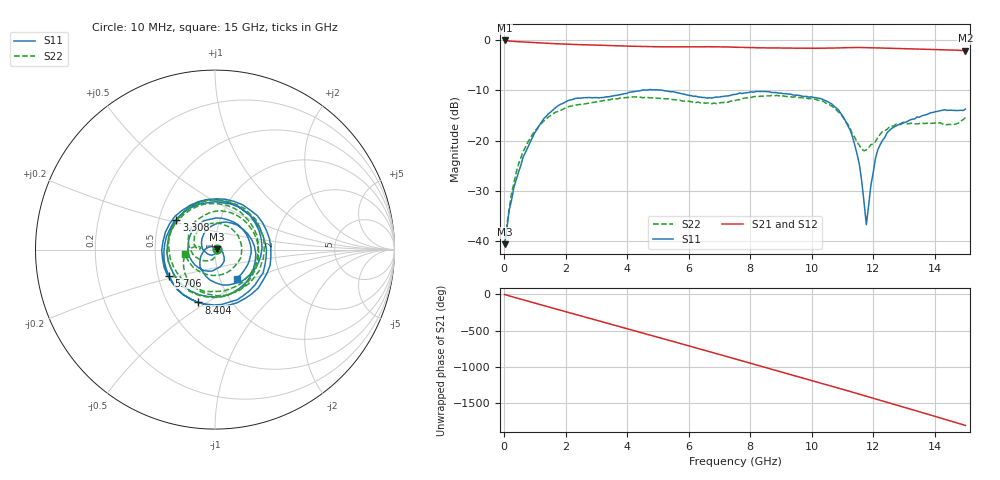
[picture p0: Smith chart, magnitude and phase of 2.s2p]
#  HZ  S  DB  R  50.00
! Rohde & Schwarz Vector Network Analyzer
! Rohde-Schwarz,ZNB3044-4Port,1351505044101548,4.21
! Created: UTC 8/5/2026, 7:53:31 PM
! freq[Hz]  db:S11  ang:S11  db:S21  ang:S21  db:S12  ang:S12  db:S22  ang:S22
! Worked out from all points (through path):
!   201 points, 10 MHz to 15 GHz, reference 50 ohm
!   highest |S21| = -0.08 dB at 10 MHz (marker M1); lowest = -2.1 dB at 15 GHz (marker M2)
!   group delay of S21, straight-line fit = 334 ps
!   lowest |S11| = -40.7 dB at 10 MHz (marker M3), VSWR 1.02, Z = 50.9 + j0.124 ohm
!   |S11| at or under -10 dB: start of sweep to 4.465 GHz; 5.153 GHz to end of sweep
!   |S22| runs from -41.0 to -11.0 dB; largest |S21 - S12| = 0.0068
!   S11 on the Smith chart (normalised r, x): 10 MHz: 1.02, +0.00; 3.308 GHz: 0.62, +0.22; 5.706 GHz: 0.57, -0.18; 8.404 GHz: 0.71, -0.46; 15 GHz: 1.20, -0.42
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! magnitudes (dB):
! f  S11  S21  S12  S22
! 10 MHz  -40.7  -0.1  -0.1  -41.0
! 159.9 MHz  -33.7  -0.2  -0.2  -33.5
! 234.8 MHz  -31.9  -0.2  -0.2  -30.5
! 459.7 MHz  -26.3  -0.3  -0.3  -24.7
! 759.5 MHz  -21.4  -0.4  -0.4  -20.4
! 1.434 GHz  -14.7  -0.7  -0.7  -15.3
! 2.558 GHz  -11.5  -0.9  -0.9  -12.7
! 3.308 GHz  -11.3  -1.1  -1.1  -12.0
! 5.032 GHz  -9.9  -1.3  -1.3  -11.6
! 5.706 GHz  -10.6  -1.3  -1.4  -11.9
! 7.505 GHz  -10.8  -1.4  -1.4  -12.0
! 8.404 GHz  -10.2  -1.6  -1.5  -11.1
! 10.05 GHz  -11.4  -1.6  -1.6  -11.7
! 10.65 GHz  -12.7  -1.6  -1.6  -13.1
! 11.25 GHz  -17.9  -1.5  -1.5  -17.6
! 11.55 GHz  -24.8  -1.5  -1.5  -20.9
! 11.78 GHz  -36.7  -1.5  -1.5  -21.8
! 11.93 GHz  -28.8  -1.5  -1.5  -20.8
! 12.08 GHz  -23.5  -1.5  -1.5  -20.2
! 12.53 GHz  -18.0  -1.6  -1.6  -17.3
! 13.88 GHz  -14.4  -1.9  -1.8  -16.6
! 15 GHz  -13.7  -2.1  -2.1  -15.4
